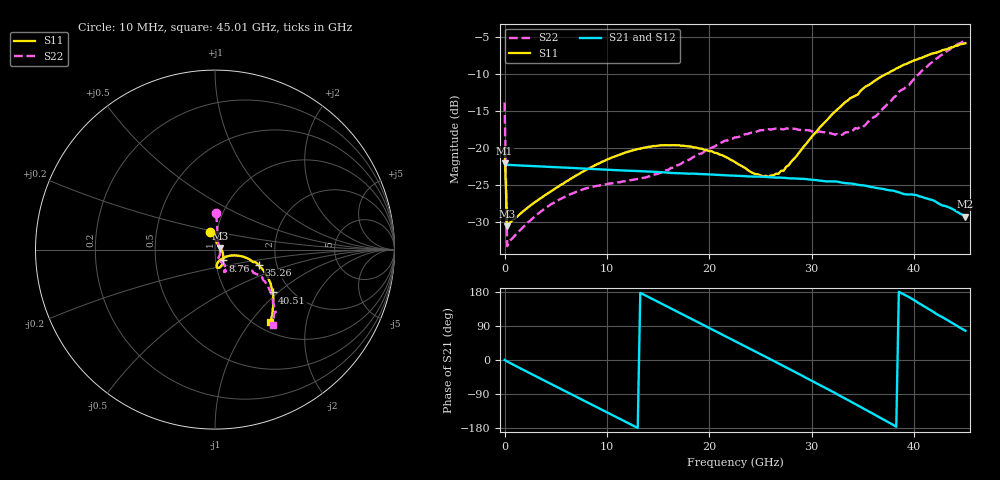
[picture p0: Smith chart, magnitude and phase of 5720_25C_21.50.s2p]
! Device:  ADRF5720
! Description: 0.5dB LSB GaAs MMIC 6-bit Digital Attenuator
! Frequency:  0.000009 -  40 GHz
! Ports:
!	RF1	= Port 1
!	RF2	= Port 2
! Vdd:  3.3 Volt
! Vss:  -3.3 Volt
! Control:  0/3.3 Volt
! State:  21.50 dB attenuation
! Data:  The device was measured using G-S-G Probes on a matrix board.
!  Data was collected using an calibrated 4 port network analyzer.
!  The reference plane for this measurement is at the launchers.
! Note:  Analog Devices supplies this data as a sample of measured data
!  for this product.  Your particular data for this product may vary.
!  Data was taken at 25 degrees C.
!  Analog Devices reserves the right to change this data at anytime.
# GHZ S DB R 45.0
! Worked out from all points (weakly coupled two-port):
!   181 points, 10 MHz to 45.01 GHz, reference 45 ohm
!   highest |S21| = -22.11 dB at 10 MHz (marker M1); lowest = -29.3 dB at 45.01 GHz (marker M2)
!   lowest |S11| = -30.6 dB at 260 MHz (marker M3), VSWR 1.06, Z = 47.6 + j0.861 ohm
!   |S11| at or under -10 dB: start of sweep to 37.36 GHz
!   |S22| runs from -33.3 to -5.5 dB; largest |S21 - S12| = 0.00012
!   S11 on the Smith chart (normalised r, x): 10 MHz: 0.93, +0.18; 8.76 GHz: 1.09, -0.13; 35.26 GHz: 1.61, -0.30; 40.51 GHz: 1.62, -0.92; 45.01 GHz: 1.15, -1.25
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0.01  -20.05 104.8  -22.11 0.1  -22.11 0.1  -13.89 88.0
0.26  -30.62 17.9  -22.30 -3.8  -22.31 -3.9  -33.28 21.9
1.26  -29.28 0.4  -22.37 -18.0  -22.37 -18.0  -31.48 -8.3
4.01  -26.35 -25.0  -22.55 -56.0  -22.55 -55.9  -28.13 -46.9
7.76  -23.14 -48.1  -22.81 -107.3  -22.81 -107.3  -25.57 -70.8
8.760001  -22.42 -52.8  -22.88 -121.0  -22.88 -121.0  -25.21 -73.4
12.01  -20.55 -65.9  -23.09 -165.5  -23.09 -165.5  -24.49 -74.5
15.26  -19.67 -76.0  -23.28 149.5  -23.28 149.5  -23.35 -66.9
19.26  -20.12 -84.1  -23.55 94.5  -23.56 94.5  -20.77 -58.9
21.51  -21.19 -84.2  -23.72 63.5  -23.73 63.5  -19.05 -59.3
22.76  -22.16 -81.3  -23.79 46.3  -23.79 46.3  -18.58 -60.1
25.26  -23.84 -60.5  -23.92 11.8  -23.92 11.8  -17.62 -63.9
26.76  -23.51 -41.6  -24.02 -8.9  -24.02 -9.0  -17.38 -65.0
27.76  -22.34 -29.4  -24.11 -23.0  -24.12 -22.9  -17.42 -66.1
30.26  -18.12 -15.2  -24.35 -58.5  -24.35 -58.5  -17.78 -65.2
32.76  -14.53 -15.1  -24.65 -94.6  -24.65 -94.5  -18.31 -55.9
35.26  -11.75 -19.6  -25.12 -131.1  -25.12 -131.2  -16.90 -39.0
37.76  -9.68 -27.3  -25.76 -168.1  -25.75 -168.1  -13.66 -29.5
40.51  -7.95 -36.6  -26.56 149.2  -26.55 149.2  -10.00 -32.2
42.26  -7.13 -42.7  -27.41 120.2  -27.40 120.2  -7.91 -38.3
43.76  -6.44 -48.0  -28.27 96.8  -28.27 96.8  -6.29 -45.7
45.01  -5.89 -52.9  -29.28 77.3  -29.28 77.4  -5.52 -52.4
